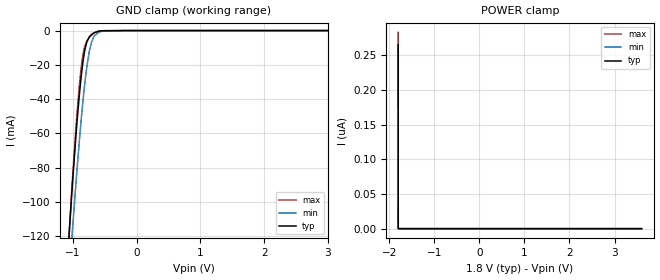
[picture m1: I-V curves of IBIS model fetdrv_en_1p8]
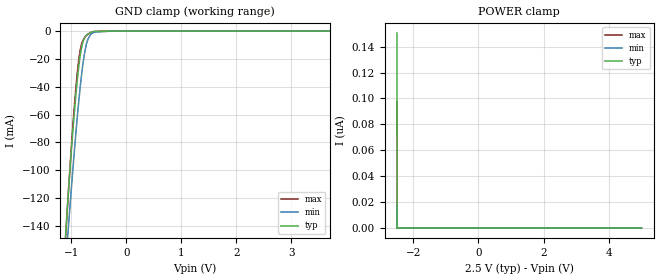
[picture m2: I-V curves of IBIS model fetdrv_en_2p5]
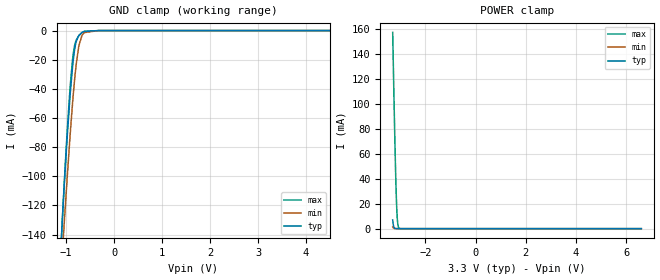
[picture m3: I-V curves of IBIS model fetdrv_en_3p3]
|Texas Instruments Incorporated
| Dual Temperature Controlled DAC with Integrated EEPROM and
| Output ON/OFF Control
| Marketing part#   Digital Voltage Range   Package-type   #pins
| LMP92066PWP   1.65V-3.6V   TSSOP   16
| LMP92066PWPR   1.65V-3.6V   TSSOP   16
[IBIS Ver]   4.1
[File name]   lmp92066.ibs
[File Rev]   1.0
[Date]   9/27/2013
[Source]
| Texas Instruments Incorporated.
| Analog-eLab Design Center, HPA
| 12500 TI Blvd
| Dallas, TX -75243
[Notes]   Revision History:
| Rev 1.0: 9/27/2013
| - Initial version of the model
| - Model generated from simulations in SPECTRE
| - Model matched to SPICE simulation
| - C_comp although listed in numerical order of value are
|   obtained from varying PVT conditions. For PVT conditions for
|   each specific value refer the buffer description under
|   respective [Model]. IBIS model user is responsible for using
|   appropriate C_comp to simulate for Signal Integrity.
|*EXCEPTION:   *
|* For sda_1p8 model, there will be leakage currents in Pulldown IV Table *
|* because of Transistors(M14) connected to the Pad.   *
[Disclaimer]
| This model is designed as an aid for customers of Texas Instruments.
| TI and its licensors and suppliers make no warranties, either expressed
| or implied, with respect to this  model, including the warranties of
| merchantability or fitness for a particular purpose. The model is
| provided solely on an "as is" basis. The entire risk as to its quality
| and performance is with the customer.
[Copyright]
(C) Copyright 2013 Texas Instruments Incorporated.All rights reserved.
|   LMP92066PWP
[Component]   LMP92066PWP
[Manufacturer]   TI
[Package]   |16 TSSOP - PWP package
| variable   typ   min   max
R_pkg   0.01   0.008   0.12
L_pkg   1.0nH   0.8nH   1.2nH
C_pkg   0.2pF   0.16pF   0.24pF
[Pin]  signal_name   model_name   R_pin   L_pin   C_pin
1   GNDD   GND   NA   NA   NA
2   DRVEN1   DRVEN   NA   NA   NA
3   DRVEN0   DRVEN   NA   NA   NA
4   VIO   POWER   NA   NA   NA
5   SDA   SDA   NA   NA   NA
6   SCL   SCL   NA   NA   NA
7   A1   NC   NA   NA   NA
8   A0   NC   NA   NA   NA
9   VSSB   POWER   NA   NA   NA
10   DAC0   NC   NA   NA   NA
11   FETDRV0   NC   NA   NA   NA
12   GNDA   GND   NA   NA   NA
13   FETDRV1   NC   NA   NA   NA
14   DAC1   NC   NA   NA   NA
15   VDDB   POWER   NA   NA   NA
16   VDD   POWER   NA   NA   NA
1000   DAP   NC   NA   NA   NA
|   Model Selectors
[Model Selector] DRVEN
fetdrv_en_1p8   1.8V  digital Input
fetdrv_en_2p5   2.5V  digital Input
fetdrv_en_3p3   3.3V  digital Input
[Model Selector] SCL
scl_1p8   1.8V  digital Input
scl_2p5   2.5V  digital Input
scl_3p3   3.3V  digital Input
[Model Selector] SDA
sda_1p8   1.8V  digital I/O_open_drain
sda_2p5   2.5V  digital I/O_open_drain
sda_3p3   3.3V  digital I/O_open_drain
| Models and submodels in the file (9): fetdrv_en_1p8 (Input), fetdrv_en_2p5 (Input), fetdrv_en_3p3 (Input), scl_1p8 (Input), scl_2p5 (Input), scl_3p3 (Input), sda_1p8 (I/O_open_drain), sda_2p5 (I/O_open_drain), sda_3p3 (I/O_open_drain)
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|   fetdrv_en_1p8 Model
[Model]   fetdrv_en_1p8
Model_type   Input
Vinl = 0.54
Vinh = 1.26
|   typ   min   max
|   (nom PVT)   (fast PVT)   (slow PVT)
C_comp   4.036e-13   3.801e-13   4.357e-13
[Model spec]
|subparameter
Vinl   0.54   0.513   0.567
Vinh   1.26   1.197   1.323
| Where nom  PVT is Nominal Process, 1.8V, 25C
|   Fast PVT is Strong Process,  1.89V, -25C
|   Slow PVT is Weak Process,   1.71V, 125C
[Voltage Range]   1.8   1.71   1.89
|Junction Temperature
[Temperature Range]   25   125   -25
[Power Clamp Reference]   1.8   1.71   1.89
[GND Clamp Reference]   0   0   0
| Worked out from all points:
|   GND clamp passes 1 mA (typ) near -0.65 V on its own axis
[GND Clamp]
|   Voltage   I(typ)   I(min)   I(max)
-1.8V     -632.4mA   -572.3mA   -659.4mA
-1.084V   -133.2mA   -156.2mA   -134.2mA
-1.01V    -90.88mA   -117.9mA   -88.47mA
-930.6mV  -51.16mA   -78.88mA   -46.04mA
-889mV    -33.71mA   -60.07mA   -28.29mA
-849.6mV  -20.27mA   -43.91mA   -15.86mA
-798.3mV  -8.92mA    -26.05mA   -7.442mA
-745.4mV  -3.904mA   -12.68mA   -4.034mA
-669.8mV  -1.322mA   -3.5mA     -1.488mA
-538mV    -102.3uA   -310.4uA   -76.66uA
-180mV    0A         0A         0A
3.6V      0A         0A         0A
[POWER Clamp]
|   Voltage   I(typ)   I(min)   I(max)
-1.8V     265.5nA    31.34nA    283nA
-1.798V   13.27nA    15.67nA    26.95nA
-1.798V   0A         14.84nA    13.48nA
-1.798V   0A         14.02nA    0A
-1.797V   0A         0A         0A
3.6V      0A         0A         0A
|   fetdrv_en_2p5 Model
[Model]   fetdrv_en_2p5
Model_type   Input
Vinl = 0.75
Vinh = 1.75
|   typ   min   max
|   (nom PVT)   (fast PVT)   (slow PVT)
C_comp   3.837e-13   3.592e-13   4.151e-13
[Model spec]
|subparameter
Vinl   0.75   0.675   0.825
Vinh   1.75   1.575   1.925
| Where nom  PVT is Nominal Process, 2.5V, 25C
|   Fast PVT is Strong Process,  2.75V, -25C
|   Slow PVT is Weak Process,   2.25V, 125C
[Voltage Range]   2.5   2.25   2.75
|Junction Temperature
[Temperature Range]   25   125   -25
[Power Clamp Reference]   2.5   2.25   2.75
[GND Clamp Reference]   0   0   0
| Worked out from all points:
|   GND clamp passes 1 mA (typ) near -0.65 V on its own axis
[GND Clamp]
|   Voltage   I(typ)   I(min)   I(max)
-2.5V     -1.154A    -1.002A    -1.199A
-1.105V   -145.9mA   -167.3mA   -147.7mA
-1.062V   -120.2mA   -144.7mA   -120.1mA
-965.5mV  -67.34mA   -95.46mA   -63.1mA
-917.5mV  -45.04mA   -72.52mA   -39.64mA
-866.5mV  -25.36mA   -50.39mA   -20.3mA
-797.7mV  -8.723mA   -25.71mA   -7.295mA
-747.2mV  -3.967mA   -12.93mA   -4.082mA
-697.7mV  -1.983mA   -5.664mA   -2.226mA
-648.2mV  -922.4uA   -2.353mA   -1.021mA
-250mV    0A         0A         0A
5V        0A         0A         0A
[POWER Clamp]
|   Voltage   I(typ)   I(min)   I(max)
-2.5V     150.6nA    17.39nA    97.6nA
-2.498V   150.1nA    12.84nA    97.36nA
-2.498V   150.1nA    12.13nA    97.33nA
-2.497V   142.6nA    11.41nA    97.3nA
-2.495V   90.05nA    0A         66.34nA
-2.495V   75.04nA    0A         57.5nA
-2.494V   60.03nA    0A         48.65nA
-2.493V   22.51nA    0A         26.54nA
-2.493V   0A         0A         13.27nA
-2.492V   0A         0A         0A
5V        0A         0A         0A
|   fetdrv_en_3p3 Model
[Model]   fetdrv_en_3p3
Model_type   Input
Vinl = 0.99
Vinh = 2.31
|   typ   min   max
|   (nom PVT)   (fast PVT)   (slow PVT)
C_comp   3.651e-13   3.429e-13   3.928e-13
[Model spec]
|subparameter
Vinl   0.99   0.9   1.08
Vinh   2.31   2.1   2.52
| Where nom  PVT is Nominal Process, 3.3V, 25C
|   Fast PVT is Strong Process,  3.6V, -25C
|   Slow PVT is Weak Process,   3V, 125C
[Voltage Range]   3.3   3   3.6
|Junction Temperature
[Temperature Range]   25   125   -25
[Power Clamp Reference]   3.3   3   3.6
[GND Clamp Reference]   0   0   0
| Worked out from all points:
|   GND clamp passes 1 mA (typ) near -0.65 V on its own axis
|   POWER clamp passes 1 mA (typ) near -3.24 V on its own axis
[GND Clamp]
|   Voltage   I(typ)   I(min)   I(max)
-3.3V     -1.755A    -1.502A    -1.822A
-1.144V   -169.5mA   -187.8mA   -173mA
-1.063V   -119.8mA   -144.4mA   -119.6mA
-1.039V   -106.3mA   -132.2mA   -105mA
-974.4mV  -71.36mA   -99.43mA   -67.36mA
-916.8mV  -44.38mA   -71.84mA   -38.92mA
-866.4mV  -25.04mA   -50mA      -19.97mA
-805.2mV  -9.732mA   -27.78mA   -7.952mA
-735mV    -3.289mA   -10.49mA   -3.505mA
-657.6mV  -1.059mA   -2.715mA   -1.176mA
-326.7mV  -338.4nA   0A         0A
6.6V      0A         0A         0A
[POWER Clamp]
|   Voltage   I(typ)   I(min)   I(max)
-3.3V     7.038mA    1.27mA     157mA
-3.28V    3.622mA    722.8uA    136mA
-3.26V    1.775mA    408.6uA    115.6mA
-3.214V   301uA      105uA      70.39mA
-3.192V   130.6uA    55.89uA    51.66mA
-3.178V   74.62uA    36.69uA    40.3mA
-3.152V   28.05uA    17.49uA    23.36mA
-3.131V   12.11uA    9.219uA    12.69mA
-3.106V   4.536uA    4.305uA    5.172mA
-3.077V   1.48uA     1.731uA    1.541mA
-3.034V   274.6nA    329.3nA    214.7uA
6.6V      0A         0A         0A
